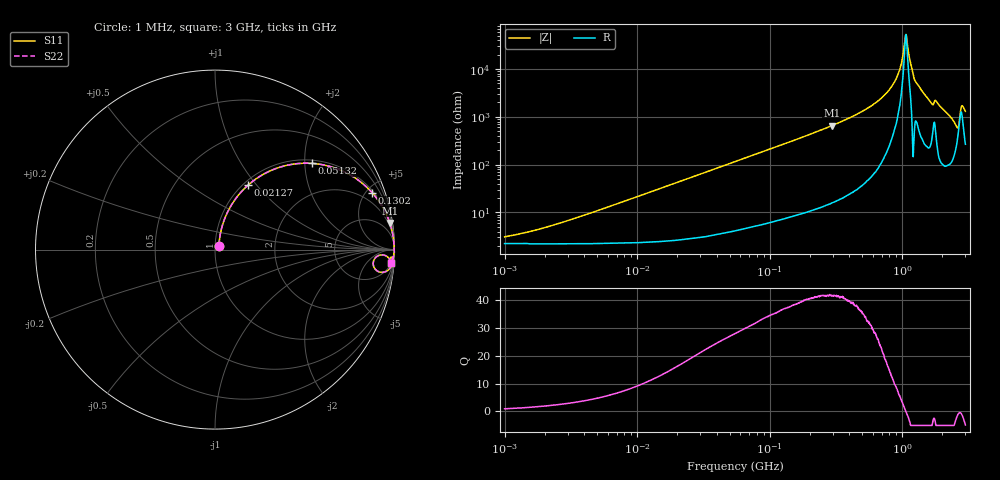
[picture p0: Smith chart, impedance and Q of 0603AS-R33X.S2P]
!s-Parameter Generated by FASTRON Sdn. Bhd.
!FASTRON P/N : 0603AS-R33X
!Keysight Technologies: E4991B_MY54100416_A.01.15
!Date created: Wed Oct 04 11:52:51 2023
!Version  : Rev01 Wed Oct 04 11:52:51 2023
!Data & Calibration Information:
!Freq	S11	S21	S12	S22
!PortZ  Port1:50+j0  Port2:50+j0
!When reading reference impedance value at option line is always used.
! Remarks : This data is being provided solely for informational purposes.
# Hz S dB R 50
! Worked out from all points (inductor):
!   1601 points, 1 MHz to 3 GHz, reference 50 ohm
!   read as one part in series: L = 339 nH near 3.114 MHz
!   highest Q = 41.6 at 294.3 MHz (marker M1), where L = 354 nH
!   self-resonance near 1.065 GHz
!   S11 on the Smith chart (normalised r, x): 1 MHz: 1.04, +0.04; 21.27 MHz: 1.05, +0.90; 51.32 MHz: 1.08, +2.16; 130.2 MHz: 1.15, +5.48; 3 GHz: 6, -26
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1000000  -30.37 42.6  -0.19 -1.2  -0.19 -1.2  -30.37 42.6
3804036  -21.72 70.1  -0.22 -4.5  -0.22 -4.5  -21.72 70.1
1.447069e7  -10.81 68.7  -0.58 -16.7  -0.58 -16.7  -10.81 68.7
2.127285e7  -7.90 62.9  -1.00 -23.7  -1.00 -23.7  -7.90 62.9
5.132264e7  -2.84 41.8  -3.52 -46.1  -3.52 -46.1  -2.84 41.8
5.477226e7  -2.58 40.0  -3.83 -47.9  -3.83 -47.9  -2.58 40.0
1.30174e8  -0.62 19.8  -9.38 -68.6  -9.38 -68.6  -0.62 19.8
2.083556e8  -0.26 12.5  -13.26 -76.0  -13.26 -76.0  -0.26 12.5
2.942768e8  -0.13 8.7  -16.44 -80.0  -16.44 -80.0  -0.13 8.7
5.528145e8  -0.04 3.7  -23.76 -84.5  -23.76 -84.5  -0.04 3.7
7.925923e8  -0.02 1.6  -31.09 -84.6  -31.09 -84.6  -0.02 1.6
9.349007e8  -0.02 0.7  -38.12 -80.8  -38.12 -80.8  -0.02 0.7
9.828732e8  -0.02 0.4  -42.06 -76.4  -42.06 -76.4  -0.02 0.4
1.0437e9  -0.02 0.1  -51.12 -48.3  -51.12 -48.3  -0.02 0.1
1.070143e9  -0.02 -0.0  -54.48 8.0  -54.48 8.0  -0.02 -0.0
1.097256e9  -0.02 -0.1  -49.94 53.5  -49.94 53.5  -0.02 -0.1
1.249715e9  -0.02 -1.0  -35.12 81.7  -35.12 81.7  -0.02 -1.0
1.637435e9  -0.06 -2.8  -26.22 80.1  -26.22 80.1  -0.06 -2.8
1.827992e9  -0.07 -2.8  -26.21 79.7  -26.21 79.7  -0.07 -2.8
2.568929e9  -0.61 -7.8  -16.60 58.7  -16.60 58.7  -0.61 -7.8
2.825159e9  -0.33 -2.4  -24.99 46.9  -24.99 46.9  -0.33 -2.4
3e9  -0.16 -4.2  -22.49 74.0  -22.49 74.0  -0.16 -4.2
